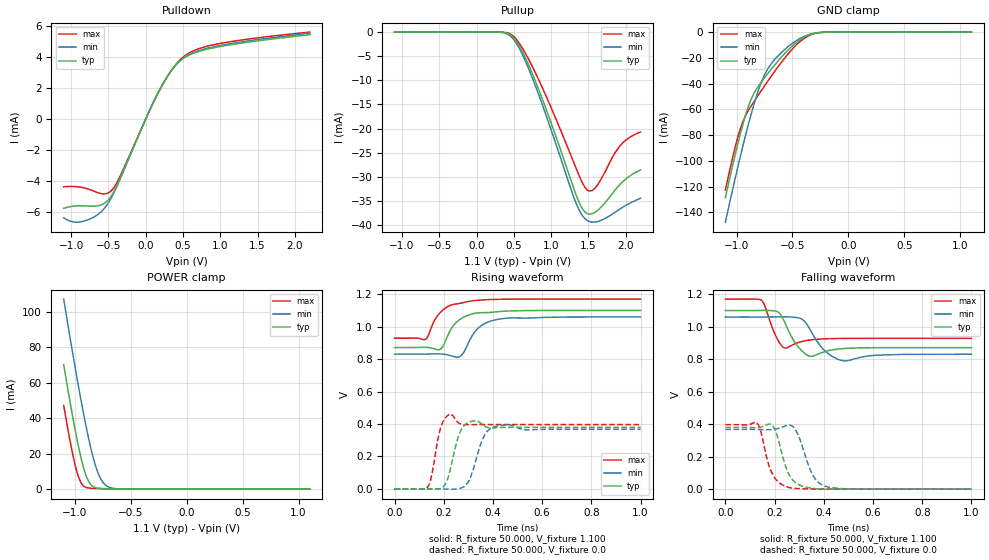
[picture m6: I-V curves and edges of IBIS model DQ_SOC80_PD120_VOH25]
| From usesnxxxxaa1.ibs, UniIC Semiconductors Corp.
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|   Model DQ_SOC80_PD120_VOH25
[Model] DQ_SOC80_PD120_VOH25
Model_type I/O
Polarity   Non-Inverting
Enable   Active-High
Vinl =  0.113V
Vinh =  0.253V
Vmeas =  0.183V
Rref =  50.000
Vref =  0.183V
C_comp   1.110pF   1.087pF   1.118pF
[Model Spec]
Vinh   0.253V   0.247V   0.265V
Vinl   0.113V   0.107V   0.125V
Vmeas   0.183V   NA   NA
Vref   0.183V   NA   NA
Rref   50.000   NA   NA
[Temperature Range]   25.000   0.125k   -40.000
[Voltage Range]   1.100V   1.060V   1.170V
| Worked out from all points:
|   slope of the pulldown table from 0 to 0.165 V, typ, clamps not added: 97.2 ohm
|   GND clamp passes 1 mA (typ) near -0.30 V on its own axis
|   POWER clamp passes 1 mA (typ) near -0.82 V on its own axis
|   rising waveform, R_fixture 50.000, V_fixture 1.100: 20-80 % time 67.5ps typ, 67.5ps min, 69.1ps max; typ from 0.871 V to 1.1 V
|   rising waveform, R_fixture 50.000, V_fixture 0.0: 20-80 % time 36.4ps typ, 45.8ps min, 27.7ps max; typ from 0 V to 0.38 V
|   falling waveform, R_fixture 50.000, V_fixture 1.100: 20-80 % time 44.5ps typ, 57.2ps min, 33.2ps max; typ from 1.1 V to 0.871 V
|   falling waveform, R_fixture 50.000, V_fixture 0.0: 20-80 % time 48.7ps typ, 54.8ps min, 46ps max; typ from 0.38 V to 0 V
[Pulldown]
|Voltage   I(typ)   I(min)   I(max)
-1.1V     -5.782mA   -6.401mA   -4.39mA
-930mV    -5.626mA   -6.683mA   -4.384mA
-760mV    -5.645mA   -6.499mA   -4.555mA
-590mV    -5.548mA   -5.975mA   -4.837mA
-454mV    -4.933mA   -5.041mA   -4.613mA
-352mV    -3.946mA   -3.975mA   -3.789mA
158mV     1.632mA    1.624mA    1.612mA
328mV     3.027mA    3.03mA     3.03mA
498mV     3.901mA    3.932mA    3.996mA
668mV     4.306mA    4.356mA    4.475mA
940mV     4.641mA    4.702mA    4.836mA
2.2V      5.457mA    5.559mA    5.628mA
[Pullup]
|Voltage   I(typ)   I(min)   I(max)
-1.1V     1nA        30.06nA    -1.059nA
296mV     -10.87uA   -31.47uA   -4.538uA
466mV     -722.3uA   -981.5uA   -506.7uA
568mV     -2.738mA   -3.216mA   -2.197mA
704mV     -7.017mA   -7.806mA   -5.798mA
942mV     -16.37mA   -17.69mA   -13.61mA
1.316V    -32.95mA   -34.73mA   -27.51mA
1.418V    -36.6mA    -38.02mA   -31.21mA
1.486V    -37.63mA   -39.06mA   -32.76mA
1.622V    -36.99mA   -39.29mA   -31.7mA
1.928V    -31.51mA   -36.62mA   -23.5mA
2.2V      -28.57mA   -34.43mA   -20.69mA
[GND_clamp]
|Voltage   I(typ)   I(min)   I(max)
-1.1V     -128.5mA   -147.6mA   -122.6mA
-1.008V   -93.62mA   -112mA     -87.95mA
-962mV    -77.6mA    -95.05mA   -73.96mA
-893mV    -57.36mA   -71.21mA   -60.7mA
-847mV    -48.01mA   -56.81mA   -54.36mA
-801mV    -41.47mA   -44.23mA   -48.33mA
-755mV    -36.02mA   -34.19mA   -42.41mA
-709mV    -30.9mA    -26.94mA   -36.63mA
-525mV    -12.67mA   -10.3mA    -15.49mA
-387mV    -3.615mA   -3.065mA   -4.419mA
-249mV    -281uA     -330.6uA   -301.3uA
1.1V      0A         0A         0A
[POWER_clamp]
|Voltage   I(typ)   I(min)   I(max)
-1.1V     70.27mA    107.3mA    47.25mA
-1.039V   47.68mA    83.93mA    25.86mA
-993mV    31.88mA    66.94mA    12.35mA
-970mV    24.65mA    58.72mA    7.262mA
-947mV    18.06mA    50.74mA    3.761mA
-901mV    7.73mA     35.71mA    987.1uA
-855mV    2.348mA    22.46mA    514uA
-809mV    697.3uA    11.94mA    396.5uA
-763mV    321uA      5.097mA    322.7uA
-717mV    213.8uA    1.813mA    258.1uA
-556mV    65.24uA    79.15uA    81.64uA
1.1V      0A         0A         0A
[Ramp]
| variable   typ   min   max
dV/dt_r   0.228/36.888p   0.221/45.592p   0.238/27.657p
dV/dt_f   0.137/44.897p   0.138/58.121p   0.145/33.391p
R_load = 50.000
[Rising Waveform]
R_fixture= 50.000
V_fixture= 1.100
V_fixture_min= 1.060
V_fixture_max= 1.170
|time   V(typ)   V(min)   V(max)
0s        871.4mV    830.8mV    928.8mV
129ps     872.4mV    831.1mV    924.6mV
181ps     857.5mV    832.1mV    1.079V
197ps     879.4mV    830.5mV    1.103V
231ps     988.3mV    819.8mV    1.134V
262ps     1.04V      812.5mV    1.142V
307ps     1.075V     920.8mV    1.157V
361ps     1.086V     1.015V     1.165V
442ps     1.095V     1.05V      1.169V
1ns       1.1V       1.06V      1.17V
[Rising Waveform]
R_fixture= 50.000
V_fixture= 0.0
V_fixture_min= 0.0
V_fixture_max= 0.0
|time   V(typ)   V(min)   V(max)
0s        2.932uV    23.8uV     546.7nV
136ps     16.14uV    73.05uV    13.45mV
186ps     2.776mV    89.55uV    369.3mV
227ps     123.3mV    -1.257mV   461.1mV
255ps     303.2mV    510uV      413.5mV
284ps     393.2mV    15.97mV    395.7mV
307ps     413.4mV    64.51mV    396mV
360ps     392.6mV    313.5mV    396.7mV
409ps     376.8mV    385.3mV    396.7mV
1ns       379.8mV    367.9mV    396.7mV
[Falling Waveform]
R_fixture= 50.000
V_fixture= 1.100
V_fixture_min= 1.060
V_fixture_max= 1.170
|time   V(typ)   V(min)   V(max)
0s        1.1V       1.06V      1.17V
146ps     1.1V       1.06V      1.164V
214ps     1.091V     1.061V     917.1mV
240ps     1.031V     1.061V     869mV
285ps     898mV      1.057V     896.6mV
331ps     826.3mV    1.016V     915.8mV
397ps     843.5mV    862.9mV    925.1mV
466ps     864mV      794.5mV    927.8mV
612ps     871mV      824.7mV    928.7mV
1ns       871.4mV    830.8mV    928.8mV
[Falling Waveform]
R_fixture= 50.000
V_fixture= 0.0
V_fixture_min= 0.0
V_fixture_max= 0.0
|time   V(typ)   V(min)   V(max)
0s        379.8mV    367.9mV    396.7mV
127ps     378.3mV    367.5mV    409.6mV
141ps     380.6mV    366.9mV    369.4mV
185ps     398.3mV    366.3mV    111.9mV
210ps     331.1mV    371.6mV    52.08mV
261ps     83.87mV    394.5mV    9.183mV
293ps     31.73mV    343.4mV    3.499mV
356ps     4.356mV    83.95mV    723uV
406ps     -18.58uV   17.78mV    206.7uV
1ns       -45.43nV   27.44uV    -2.378uV
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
